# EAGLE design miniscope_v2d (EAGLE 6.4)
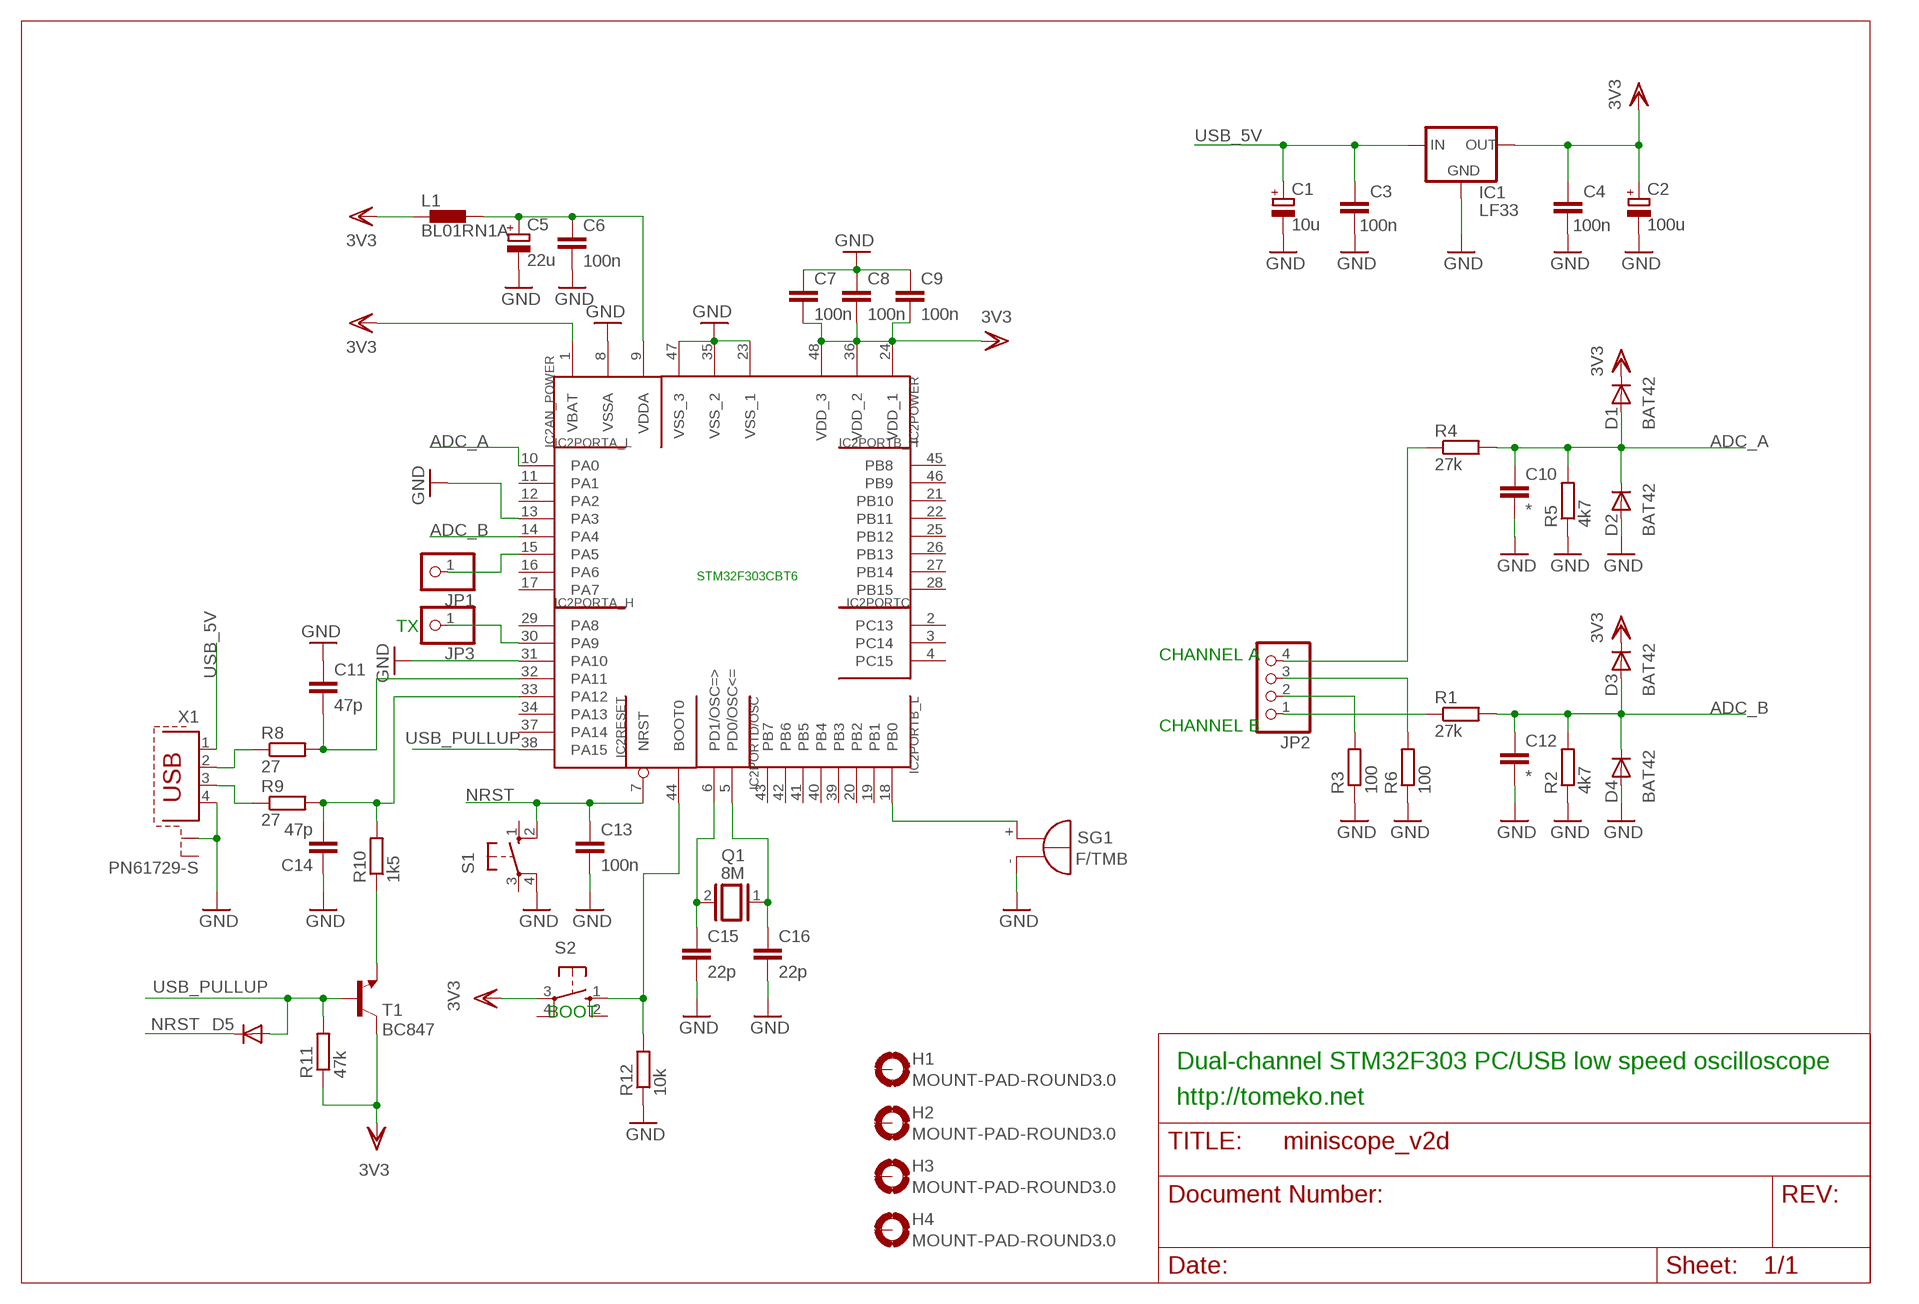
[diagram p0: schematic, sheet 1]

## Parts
C1  10u  CPOL-EUE2.5-5  [E2,5-5]
C2  100u  CPOL-EUE2.5-6  [E2,5-6]
C3  100n  C-EUC0805K  [C0805K]
C4  100n  C-EUC0805K  [C0805K]
C5  22u  CPOL-EUE2.5-5  [E2,5-5]
C6  100n  C-EUC0805K  [C0805K]
C7  100n  C-EUC0805K  [C0805K]
C8  100n  C-EUC0805K  [C0805K]
C9  100n  C-EUC0805K  [C0805K]
C10  *  C-EUC0805K  [C0805K]
C11  47p  C-EUC0805K  [C0805K]
C12  *  C-EUC0805K  [C0805K]
C13  100n  C-EUC0805K  [C0805K]
C14  47p  C-EUC0805K  [C0805K]
C15  22p  C-EUC0805K  [C0805K]
C16  22p  C-EUC0805K  [C0805K]
D1  BAT42  1N4148DO35-7  [DO35-7]
D2  BAT42  1N4148DO35-7  [DO35-7]
D3  BAT42  1N4148DO35-7  [DO35-7]
D4  BAT42  1N4148DO35-7  [DO35-7]
D5  DIODE-SOD80C  [SOD80C]
H1  MOUNT-PAD-ROUND3.0  [3,0-PAD]
H2  MOUNT-PAD-ROUND3.0  [3,0-PAD]
H3  MOUNT-PAD-ROUND3.0  [3,0-PAD]
H4  MOUNT-PAD-ROUND3.0  [3,0-PAD]
IC1  LF33  LFXXCV  [DPACK_1]
IC2  STM32F303CBT6  STM32F10XCXT6  [TQFP48]
JP1  PINHD-1X1  [1X01]
JP2  PINHD-1X4  [1X04]
JP3  PINHD-1X1  [1X01]
L1  BL01RN1A  [BL01RN1A]
Q1  8M  XTAL/S  [QS]
R1  27k  R-EU_R0805  [R0805]
R2  4k7  R-EU_R0805  [R0805]
R3  100  R-EU_R0805  [R0805]
R4  27k  R-EU_R0805  [R0805]
R5  4k7  R-EU_R0805  [R0805]
R6  100  R-EU_R0805  [R0805]
R8  27  R-EU_R0805  [R0805]
R9  27  R-EU_R0805  [R0805]
R10  1k5  R-EU_R0805  [R0805]
R11  47k  R-EU_R0805  [R0805]
R12  10k  R-EU_R0805  [R0805]
S1  10-XX  [B3F-10XX]
S2  10-XX  [B3F-10XX]
SG1  F/TMB  [F/TMB]
T1  BC847  [SOT23]
X1  PN61729-S  [PN61729-S]

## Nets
ADC_A: C10.1 D1.A D2.C IC2.10(PORTA_L:PA0) R4.2 R5.2
ADC_B: C12.1 D3.A D4.C IC2.14(PORTA_L:PA4) R1.2 R2.2
GND: C1.- C2.- C3.1 C4.1 C5.- C6.2 C7.1 C8.1 C9.1 C10.2 C11.1 C12.2 C13.2 C14.1 C15.2 C16.2 D2.A D4.A IC1.C(GND) IC2.8(AN_POWER:VSSA) IC2.13(PORTA_L:PA3) IC2.23(POWER:VSS_1) IC2.31(PORTA_H:PA10) IC2.35(POWER:VSS_2) IC2.47(POWER:VSS_3) R2.1 R3.1 R5.1 R6.1 R12.1 S1.4(P1) SG1.- X1.4 X1.S1
N$1: IC2.44(RESET:BOOT0) R12.2 S2.1(S)
N$2: C5.+ C6.1 IC2.9(AN_POWER:VDDA) L1.2
N$3: JP2.2 R3.2
N$4: R10.1 T1.2(E)
N$5: R8.1 X1.2
N$6: R9.1 X1.3
N$7: C14.2 IC2.33(PORTA_H:PA12) R9.2 R10.2
N$8: C11.2 IC2.32(PORTA_H:PA11) R8.2
N$9: IC2.30(PORTA_H:PA9) JP3.1
N$10: JP2.3 R6.2
N$11: JP2.4 R4.1
N$12: JP2.1 R1.1
N$13: IC2.15(PORTA_L:PA5) JP1.1
N$14: C16.1 IC2.5(PORTD/OSC:PD0/OSC<=) Q1.1
N$15: IC2.18(PORTB_L:PB0) SG1.+
N$37: C15.1 IC2.6(PORTD/OSC:PD1/OSC=>) Q1.2
NRST: C13.1 D5.C IC2.7(RESET:NRST) S1.2(S1)
USB_5V: C1.+ C3.2 IC1.B(IN) X1.1
USB_PULLUP: D5.A IC2.38(PORTA_H:PA15) R11.2 T1.1(B)
VDD: C2.+ C4.2 C7.2 C8.2 C9.2 D1.C D3.C IC1.E(OUT) IC2.1(AN_POWER:VBAT) IC2.24(POWER:VDD_1) IC2.36(POWER:VDD_2) IC2.48(POWER:VDD_3) L1.1 R11.1 S2.3(P) T1.3(C) ; supply symbol labelled 3V3
Unconnected: H1.B3,0(MOUNT) H2.B3,0(MOUNT) H3.B3,0(MOUNT) H4.B3,0(MOUNT) IC2.2(PORTC:PC13) IC2.3(PORTC:PC14) IC2.4(PORTC:PC15) IC2.11(PORTA_L:PA1) IC2.12(PORTA_L:PA2) IC2.16(PORTA_L:PA6) IC2.17(PORTA_L:PA7) IC2.19(PORTB_L:PB1) IC2.20(PORTB_L:PB2) IC2.21(PORTB_H:PB10) IC2.22(PORTB_H:PB11) IC2.25(PORTB_H:PB12) IC2.26(PORTB_H:PB13) IC2.27(PORTB_H:PB14) IC2.28(PORTB_H:PB15) IC2.29(PORTA_H:PA8) IC2.34(PORTA_H:PA13) IC2.37(PORTA_H:PA14) IC2.39(PORTB_L:PB3) IC2.40(PORTB_L:PB4) IC2.41(PORTB_L:PB5) IC2.42(PORTB_L:PB6) IC2.43(PORTB_L:PB7) IC2.45(PORTB_H:PB8) IC2.46(PORTB_H:PB9) S1.1(S) S1.3(P) S2.2(S1) S2.4(P1) X1.S2

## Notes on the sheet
- TX
- CHANNEL A
- CHANNEL B
- BOOT
- Dual-channel STM32F303 PC/USB low speed oscilloscope
- http://tomeko.net

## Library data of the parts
C1 C2 C5 = resistor:CPOL-EU: POLARIZED CAPACITOR, European symbol
C3 C4 C6-C16 = resistor:C-EU: CAPACITOR, European symbol
D1-D4 = diode:1N4148: DIODE
D5 = diode:DIODE-: DIODE
H1-H4 = holes:MOUNT-PAD-ROUND: MOUNTING PAD, round
IC1 = lf33:LFXXCV: VOLTAGE REGULATOR
IC2 = stm32:STM32F10XCXT6: ST STM32F101/103 48pin LQFP
JP1 JP3 = pinhead:PINHD-1X1: PIN HEADER
JP2 = pinhead:PINHD-1X4: PIN HEADER
L1 = inductors:BL0: Noise Suppression Products/EMI Suppression Filters, Lead EMIFIL(R) Inductor Type
Q1 = special:XTAL/S: CRYSTAL
R1-R6 R8-R12 = rcl:R-EU_: RESISTOR, European symbol
S1 S2 = switch-omron:10-XX: OMRON SWITCH; MPN: B3F-1000; OC_FARNELL: 176432; OC_NEWARK: 36M3542
SG1 = buzzer:F/TMB: BUZZER; OC_FARNELL: unknown; OC_NEWARK: unknown
T1 = transistor-neu-to92:BC847: NPN TRANSISTOR
X1 = con-berg:PN61729-S: BERG USB connector; OC_FARNELL: unknown; OC_NEWARK: unknown

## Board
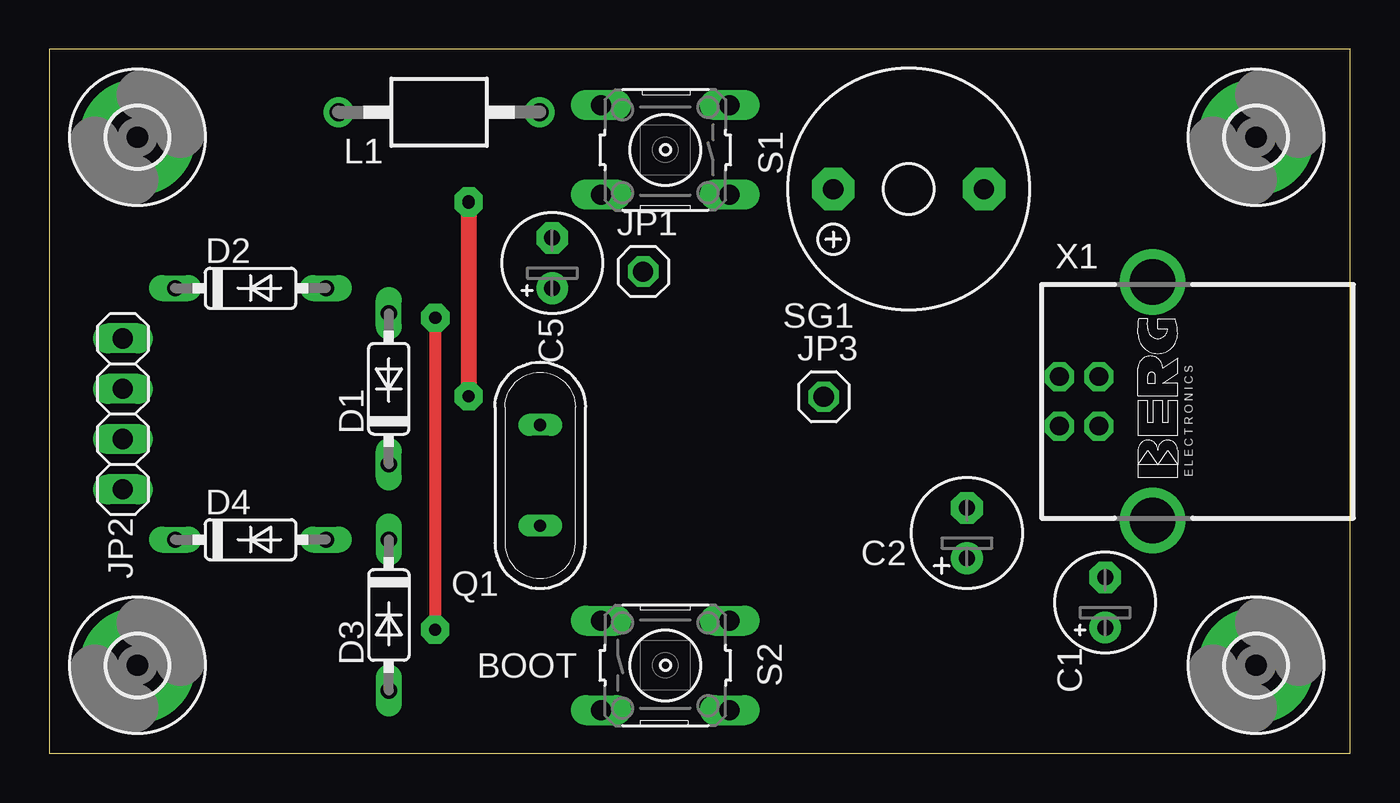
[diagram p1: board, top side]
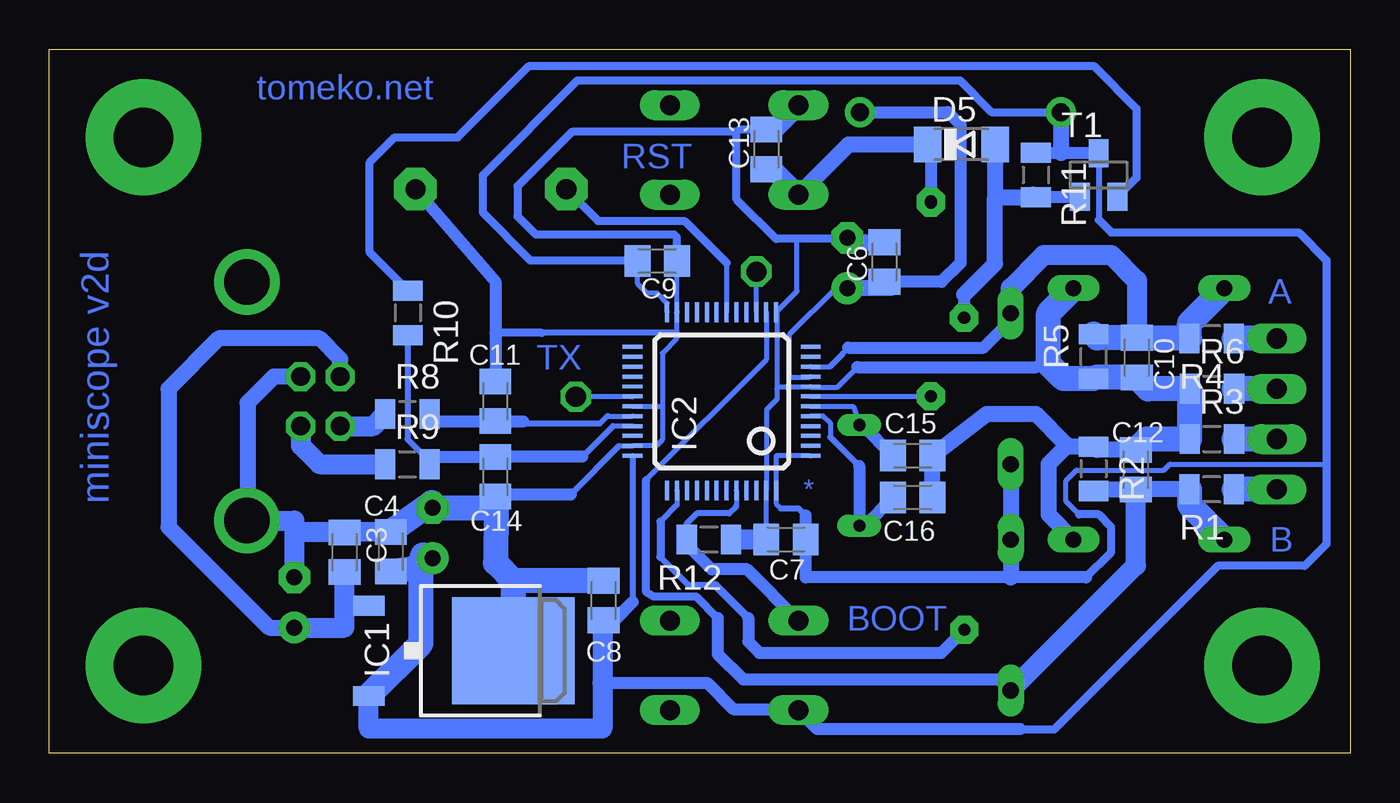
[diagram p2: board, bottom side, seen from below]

Size 65.71 x 35.55 mm. Coordinates in mm from the lower left corner, seen from the top.
Outline: 0,0 65.71,0 65.71,35.55 0,35.55 0,0
Copper layers (1*16): Top 0.035mm / dielectric 1.5mm / Bottom 0.035mm
Design rules "default": minimum track width 10mil, minimum drill 24mil, track to track 8mil, track to pad 8mil, pad to pad 8mil, via to via 8mil, smd to smd 8mil, copper to edge 40mil, drill to drill 8mil, minimum pad ring 10mil, minimum via ring 8mil, stop-mask expansion 4mil, vias tented up to drill 0mil, thermal gap 10mil

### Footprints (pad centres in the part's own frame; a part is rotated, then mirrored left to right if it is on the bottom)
E2,5-5 = drill 0.813 pad 1.6: + -1.27,0 | drill 0.813 pad 1.6 octagon: - 1.27,0
E2,5-6 = drill 0.813 pad 1.6: + -1.27,0 | drill 0.813 pad 1.6 octagon: - 1.27,0
C0805K = smd 1.3 x 1.6: 1 -1,0; 2 1,0
DO35-7 = drill 0.813 long: A 3.81,0; C -3.81,0
SOD80C = smd 1.4 x 1.8: A 1.7,0; C -1.7,0
3,0-PAD = drill 3 pad 5.842: B3,0 0,0
DPACK_1 = smd 1 x 1.6: B -2.28,-4.8; E 2.28,-4.8 | smd 5.4 x 6.2: C 0,2.5
TQFP48 = smd 0.2 x 1: 1 -2.75,-4.5; 2 -2.25,-4.5; 3 -1.75,-4.5; 4 -1.25,-4.5; 5 -0.75,-4.5; 6 -0.25,-4.5; 7 0.25,-4.5; 8 0.75,-4.5; 9 1.25,-4.5; 10 1.75,-4.5; 11 2.25,-4.5; 12 2.75,-4.5; 25 2.75,4.5; 26 2.25,4.5; 27 1.75,4.5; 28 1.25,4.5; 29 0.75,4.5; 30 0.25,4.5; 31 -0.25,4.5; 32 -0.75,4.5; 33 -1.25,4.5; 34 -1.75,4.5; 35 -2.25,4.5; 36 -2.75,4.5 | smd 1 x 0.2: 13 4.5,-2.75; 14 4.5,-2.25; 15 4.5,-1.75; 16 4.5,-1.25; 17 4.5,-0.75; 18 4.5,-0.25; 19 4.5,0.25; 20 4.5,0.75; 21 4.5,1.25; 22 4.5,1.75; 23 4.5,2.25; 24 4.5,2.75; 37 -4.5,2.75; 38 -4.5,2.25; 39 -4.5,1.75; 40 -4.5,1.25; 41 -4.5,0.75; 42 -4.5,0.25; 43 -4.5,-0.25; 44 -4.5,-0.75; 45 -4.5,-1.25; 46 -4.5,-1.75; 47 -4.5,-2.25; 48 -4.5,-2.75
1X01 = drill 1.016 octagon: 1 0,0
1X04 = drill 1.016 long: 1 -3.81,0; 2 -1.27,0; 3 1.27,0; 4 3.81,0
BL01RN1A = drill 0.9 pad 1.5: 1 -5.08,0; 2 5.08,0
QS = drill 0.61 long: 1 -2.54,0; 2 2.54,0
R0805 = smd 1.016 x 1.5: 1 -1.118,0; 2 1.128,0
B3F-10XX = drill 1.016 long: 1 -3.251,2.261; 2 3.251,2.261; 3 -3.251,-2.261; 4 3.251,-2.261
F/TMB = drill 1.016 pad 2.159 octagon: + 3.81,0; - -3.81,0
SOT23 = smd 1 x 1.4: 1 -0.95,-1.1; 2 0.95,-1.1; 3 0,1.1
PN61729-S = drill 0.95 octagon: 1 1.25,4.71; 2 -1.25,4.71; 3 -1.25,2.71; 4 1.25,2.71 | drill 2.3 pad 2.9: S1 -6.02,0; S2 6.02,0

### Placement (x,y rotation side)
C1  53.34,7.62 90 top
C2  46.35,11.13 90 top
C3  50.8,10.16 270 bottom
C4  48.46,10.19 270 bottom
C5  25.4,24.77 90 top
C6  23.52,24.82 90 bottom
C7  28.5,10.79 0 bottom
C8  37.72,7.72 270 bottom
C9  35,24.87 180 bottom
C10  10.77,19.99 270 bottom
C11  43.18,17.78 270 bottom
C12  10.82,14.33 90 bottom
C13  29.49,30.51 90 bottom
C14  43.18,13.97 90 bottom
C15  22.1,15.04 0 bottom
C16  22.1,12.93 0 bottom
D1  17.14,18.41 90 top
D2  10.16,23.5 0 top
D3  17.14,6.99 270 top
D4  10.16,10.79 0 top
D5  19.63,30.76 0 bottom
H1  60.96,4.45 0 top
H2  60.96,31.11 0 top
H3  4.45,31.11 0 top
H4  4.45,4.45 0 top
IC1  44.78,5.18 270 bottom
IC2  31.75,17.78 90 bottom
JP1  30,24.33 0 top
JP2  3.71,17.14 90 top
JP3  39.12,18.01 0 top
L1  19.68,32.38 0 top
Q1  24.79,14.05 90 top
R1  6.99,13.34 180 bottom
R2  12.95,14.38 270 bottom
R3  6.99,15.88 0 bottom
R4  6.99,20.95 180 bottom
R5  12.95,20.04 90 bottom
R6  6.99,18.41 0 bottom
R8  47.62,17.14 0 bottom
R9  47.62,14.61 0 bottom
R10  47.6,22.25 270 bottom
R11  15.88,29.21 270 bottom
R12  32.38,10.79 180 bottom
S1  31.11,30.48 180 top
S2  31.11,4.45 0 top
SG1  43.41,28.5 180 top
T1  12.7,29.21 0 bottom
X1  55.73,17.78 90 top

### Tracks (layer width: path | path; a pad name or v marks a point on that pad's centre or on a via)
ADC_A
  Bottom 0.254: IC2.10 26.29,19.53 | 25.63,20.19 25.63,20.22 25.35,20.5
  Bottom 0.305: 26.29,19.53 25.63,20.19
  Bottom 0.61: 25.35,20.5 18.52,20.5 17.14,21.87 D1.A
  Bottom 1.016: D1.A 17.14,23.5 15.47,25.17 12.06,25.17 10.77,23.88 C10.1
  Bottom 1.27: R5.2 12.78,20.99 C10.1 10.73,20.95 R4.2 8.11,21.73 D2.C
ADC_B
  Bottom 0.254: IC2.14 29.46,22.25 29.46,19.91 35.56,13.82
  Bottom 0.406: 35.56,13.82 35.56,8.15 35.18,7.92 33.05,7.92 31.95,6.83
  Bottom 0.61: 31.95,6.83 31.95,5.03 30.66,3.73 17.7,3.73 D3.A
  Bottom 0.813: R1.2 10.79,13.34 12.87,13.34 R2.2 12.88,13.33 C12.1
  Bottom 1.016: D3.A 10.82,9.5 C12.1
  Bottom 1.27: 10.79,13.34 C12.1 | R1.2 8.11,12.56 D4.C
GND
  Bottom 0.254: C7.1 IC2.47 29.46,13.31 29.46,17.37 28.96,17.88 28.96,18.41 | 37.26,9.18 C8.1 | 34.14,26.21 34.04,26.11 | 30.89,31.5 30.99,31.39 | 34.04,24.89 C9.1 IC2.23 34.04,22.25 34.04,21.23 34.04,20.93 34.75,20.22 34.75,17.53 | 29.97,31.5 C13.2 | C5.- 24.82,26.01 24.84,25.98 | 24.89,19.51 25.91,18.49 27.23,18.49 IC2.8 27.33,18.49 28.88,18.49 28.96,18.41 | 15.85,19.51 15.24,19.68 | 34.75,17.53 34.75,15.85 35.05,15.54 36.17,15.54 IC2.35 36.92,15.53 | 43.18,18.8 C11.1 | C14.1 43.07,13.08 | IC2.31 34.75,17.53 | 27.94,25.98 27.94,23.34 IC2.13 28.96,22.25 28.96,18.41
  Bottom 0.305: 34.04,21.23 40.84,21.23 | 39.37,13.08 36.92,15.53
  Bottom 0.406: 34.04,26.11 34.04,24.89 | 34.14,26.21 41.15,26.21 42.06,27.13 42.06,28.65 39.32,31.39 30.99,31.39 30.99,27.97 29,25.98 27.94,25.98 24.84,25.98 | 29.97,31.5 30.89,31.5 | 40.84,21.23 43.18,21.23
  Bottom 0.61: 24.89,19.51 15.85,19.51 | C11.1 43.18,21.23 43.18,23.82 SG1.- | 43.07,13.08 39.37,13.08
  Bottom 0.813: C12.2 12.79,15.33 R2.1 14.35,15.49 | 14.35,15.49 15.24,14.61 15.24,12.06 D4.A | X1.4 54.38,19.03 55.7,17.7 55.7,11.79 X1.S1 | C16.2 C15.2 18.36,17.14 15.88,17.14 14.35,15.62 14.35,15.49 | C5.- 24.55,25.82 C6.2
  Bottom 1.016: 51.03,11.16 53.34,11.16 | 53.34,11.16 C1.- | X1.S1 53.34,11.76 53.34,11.16 | S1.4 29.1,31.5 C13.2 | C7.1 R12.1 arc-90 R12.1 31.11,10.79 | C4.1 51.03,11.16 | 51.03,11.16 C3.1
  Bottom 1.27: C12.2 10.27,15.88 R3.1 R6.1 10.2,18.41 C10.2 12.89,18.99 R5.1 14.48,18.92 15.24,19.68 15.24,22.23 D2.A | C4.1 46.4,12.66 C2.- 43.16,12.39 | C8.1 42.28,8.72 | 42.28,8.72 IC1.C | C14.1 43.16,12.39 | 43.16,12.39 43.18,9.62 42.28,8.72
N$1
  Bottom 0.254: IC2.44 31,12.48
  Bottom 0.305: 31,12.48 31.37,12.12 32.99,12.12 33.51,11.6 R12.2
  Bottom 0.61: S2.1 30.45,9.3 32.26,9.3 33.51,10.55 R12.2
N$2
  Bottom 0.254: 26.01,23.47 28.35,21.13 28.35,19.1 28.25,19 27.33,19 IC2.9 | 24.18,23.47 C5.+
  Bottom 0.406: 24.18,23.47 26.01,23.47
  Bottom 0.61: L1.2 20.32,32.38 19.68,31.75 19.68,24.77 20.63,23.82 C6.1
  Bottom 0.813: C6.1 23.21,23.5 C5.+
N$3
  Bottom 1.27: JP2.2 R3.2
N$4
  Bottom 0.406: R10.1 49.53,25.3 49.53,29.84 48.26,31.11 45.09,31.11 41.48,34.72 12.95,34.72 10.79,32.56 10.79,29.07 T1.2
N$5
  Bottom 1.016: X1.2 49.36,16.53 R8.1
N$6
  Bottom 1.016: X1.3 53.02,15.55 52.07,14.61 R9.1
N$7
  Bottom 0.254: IC2.33 37.24,16.53 | 43.16,14.99 C14.2
  Bottom 0.305: 37.24,16.53 38.79,14.99 | R10.2 47.62,21.1 47.62,15.88 46.5,14.75 R9.2
  Bottom 0.61: R9.2 46.13,14.97 C14.2 | 38.79,14.99 43.16,14.99
N$8
  Bottom 0.254: 37.9,16.66 37.49,17.07 37.45,17.03 IC2.32 | 41.76,16.76 41.66,16.66 | 42.98,16.76 C11.2
  Bottom 0.305: 41.66,16.66 37.9,16.66
  Bottom 0.61: R8.2 46.13,16.78 C11.2 | 42.98,16.76 41.76,16.76
N$9
  Bottom 0.254: IC2.30 36.27,18.01 JP3.1
N$10
  Bottom 1.27: JP2.3 R6.2
N$11
  Bottom 1.27: JP2.4 R4.1
N$12
  Bottom 1.27: JP2.1 R1.1
N$13
  Bottom 0.254: IC2.15 JP1.1
N$14
  Bottom 0.254: IC2.5 27.24,17.04 26.62,17.04 26.26,16.69 26.26,15.98
  Bottom 0.305: 26.26,15.98 24.79,14.5
  Bottom 0.61: 24.79,14.5 Q1.1 24.52,11.51 C16.1
N$15
  Bottom 0.254: 31.5,24.77 IC2.18
  Bottom 0.406: SG1.+ 38,26.9 33.63,26.9 31.5,24.77
N$16  (via drill 0.6 pad 1.42)
  other vias: 21.18,27.81
N$17  (via drill 0.6 pad 1.42)
  other vias: 19.48,22
N$37
  Bottom 0.254: IC2.6 25.1,17.53 Q1.2
  Bottom 0.61: C15.1 24.65,16.59 Q1.2
NRST  (via drill 0.6 pad 1.42)
  Top 0.813: v21.18,27.89 v21.18,18.03
  Bottom 0.254: IC2.7 v21.18,18.03
  Bottom 0.61: D5.C 21.18,30.61 v21.18,27.89
  Bottom 0.813: S1.2 25.32,30.76 D5.C
  Bottom 1.016: S1.2 29.15,29.5 C13.1
USB_5V
  Bottom 0.813: X1.1 51.02,19.9 52.07,20.95 57.15,20.95 59.69,18.41 59.69,11.43 54.61,6.35 C1.+
  Bottom 1.016: IC1.B 50.8,7.46 | 50.8,7.46 C3.2 | C1.+ 50.8,6.35 50.8,7.46
USB_PULLUP  (via drill 0.6 pad 1.42)
  Top 0.61: v19.51,22 19.48,21.97 v19.48,6.25
  Bottom 0.254: IC2.38 34.01,13.27 34.01,12.55
  Bottom 0.305: 34.01,12.55 34.85,11.71 | 34.85,9.91 33.45,8.51 32.08,8.51
  Bottom 0.406: 34.85,11.71 34.85,9.91 | 32.08,8.51 30.4,6.83
  Bottom 0.61: T1.1 13.68,28.08 R11.2 | 19.51,23.16 v19.51,22 | 30.4,6.83 30.4,5.64 29.84,5.08 20.65,5.08 v19.48,6.25
  Bottom 0.813: 16.01,28.22 R11.2 17.93,28.08 | D5.A 17.93,28.08 | 19.51,23.16 17.93,24.74 17.93,28.08
VDD
  Bottom 0.254: IC2.24 34.5,22.74 35,23.24 35.51,23.24 35.99,23.72 35.99,24.86 C9.2 35.97,24.89 | 28.75,12.37 29,12.62 IC2.48 29,15.03 IC2.1 | 27.51,10.8 C7.2 | C8.2 37.17,6.72 | 27.94,2.23 S2.3 27.84,2.13 | 36.25,7.65 36.25,7.64 | 13.69,12.06 14.35,12.72 14.35,13.77 13.82,14.3 9.4,14.3 9.09,14.61 1.19,14.61
  Bottom 0.305: 28.75,12.37 27.86,12.37 27.51,12.01 | IC2.36 36.25,7.65 | T1.3 12.7,26.95 | 16.64,1.19 16.66,1.22
  Bottom 0.406: 35.97,24.89 41.43,24.89 41.43,24.92 43.81,27.3 43.81,29.21 39.04,33.98 19.71,33.98 18.11,32.38 L1.1 | 12.7,26.95 12.06,26.31 2.59,26.31 1.19,24.92 1.19,14.61 1.19,10.57 2.29,9.47 6.68,9.47 14.96,1.19 16.64,1.19 | 13.34,8.89 12.06,10.16 12.06,11.43 12.7,12.06 13.69,12.06
  Bottom 0.61: 27.51,12.01 27.51,10.8 | T1.3 14.61,30.31 15.86,30.31 R11.1 | 27.94,2.23 31.17,2.23 32.49,3.56 37.77,3.56 | 27.84,2.13 26.92,1.22 16.66,1.22 | 36.25,7.64 37.17,6.72 | 13.34,8.89 17.14,8.89 27.5,8.89 C7.2
  Bottom 0.813: L1.1 14.61,30.31 | 17.14,8.89 D3.C D1.C
  Bottom 1.016: C8.2 37.77,6.67 37.77,3.56 37.77,1.25 49.58,1.25 IC1.E
  Bottom 1.27: C4.2 46.94,9.39 | 46.94,9.39 46.85,10.02 C2.+ | IC1.E 46.94,5.54 46.94,9.39

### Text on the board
Bottom: tomeko.net | RST | miniscope v2d | A | TX | * | B | BOOT
tNames: BOOT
